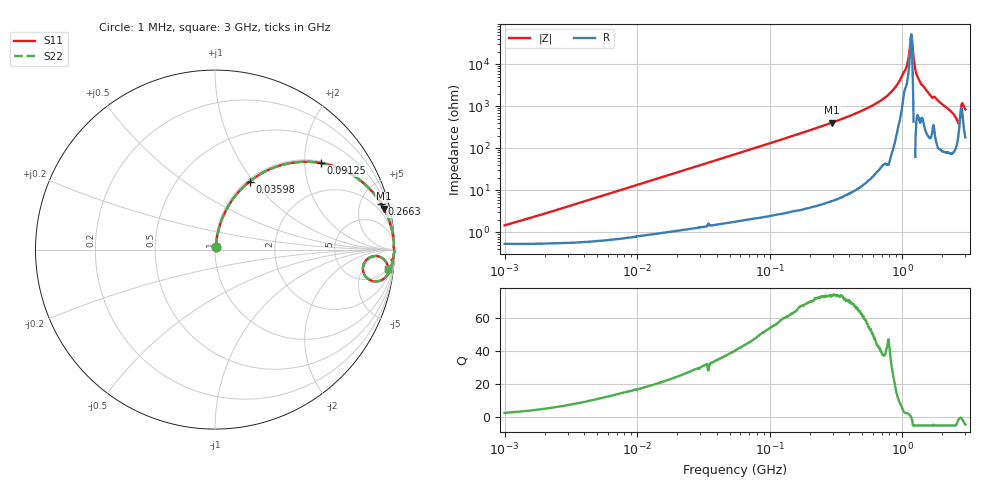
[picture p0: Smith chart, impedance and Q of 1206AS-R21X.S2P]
!s-Parameter Generated by FASTRON Sdn. Bhd.
!FASTRON P/N : 1206AS-R21X
!Keysight Technologies: E4991B_MY54100416_A.01.15
!Date created: Thu Nov 16 10:02:58 2023
!Version  : Rev00 Thu Nov 16 10:02:58 2023
!Data & Calibration Information:
!Freq	S11	S21	S12	S22
!PortZ  Port1:50+j0  Port2:50+j0
!When reading reference impedance value at option line is always used.
! Remarks : This data is being provided solely for informational purposes.
# Hz S dB R 50
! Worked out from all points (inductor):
!   1601 points, 1 MHz to 3 GHz, reference 50 ohm
!   read as one part in series: L = 219 nH near 1.168 MHz
!   highest Q = 73.5 at 295.8 MHz (marker M1), where L = 221 nH
!   self-resonance near 1.165 GHz
!   S11 on the Smith chart (normalised r, x): 1 MHz: 1.01, +0.03; 35.98 MHz: 1.03, +0.95; 91.25 MHz: 1.05, +2.41; 266.3 MHz: 1.10, +7.31; 3 GHz: 5, -16
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1000000  -36.66 67.9  -0.05 -0.8  -0.05 -0.8  -36.66 67.9
3804036  -25.68 80.6  -0.06 -3.0  -0.06 -3.0  -25.68 80.6
1.447069e7  -14.46 76.3  -0.24 -10.9  -0.24 -10.9  -14.46 76.3
3.597591e7  -7.42 63.1  -0.99 -25.2  -0.99 -25.2  -7.42 63.1
5.477226e7  -4.74 53.2  -1.93 -35.4  -1.93 -35.4  -4.74 53.2
9.124879e7  -2.36 39.3  -3.97 -49.6  -3.97 -49.6  -2.36 39.3
2.083556e8  -0.56 19.5  -9.52 -69.6  -9.52 -69.6  -0.56 19.5
2.662515e8  -0.34 15.2  -11.60 -74.0  -11.60 -74.0  -0.34 15.2
2.957531e8  -0.28 13.6  -12.55 -75.6  -12.55 -75.6  -0.28 13.6
5.473095e8  -0.07 6.3  -19.26 -82.7  -19.26 -82.7  -0.07 6.3
7.925923e8  -0.02 3.0  -25.73 -85.8  -25.73 -85.8  -0.02 3.0
1.0437e9  -0.04 0.8  -36.89 -69.0  -36.89 -69.0  -0.04 0.8
1.091779e9  -0.03 0.5  -40.09 -66.7  -40.09 -66.7  -0.03 0.5
1.142072e9  -0.02 0.2  -47.64 -50.3  -47.64 -50.3  -0.02 0.2
1.171007e9  -0.02 -0.0  -54.23 5.0  -54.23 5.0  -0.02 -0.0
1.200675e9  -0.01 -0.2  -47.88 76.2  -47.88 76.2  -0.01 -0.2
1.262285e9  -0.00 -0.8  -36.93 87.7  -36.93 87.7  -0.00 -0.8
1.313842e9  -0.02 -1.2  -33.81 81.8  -33.81 81.8  -0.02 -1.2
1.629261e9  -0.06 -3.1  -25.38 81.5  -25.38 81.5  -0.06 -3.1
2.607784e9  -0.73 -11.1  -13.88 61.2  -13.88 61.2  -0.73 -11.1
2.853575e9  -0.42 -3.9  -21.74 52.9  -21.74 52.9  -0.42 -3.9
3e9  -0.28 -6.4  -18.79 71.1  -18.79 71.1  -0.28 -6.4
